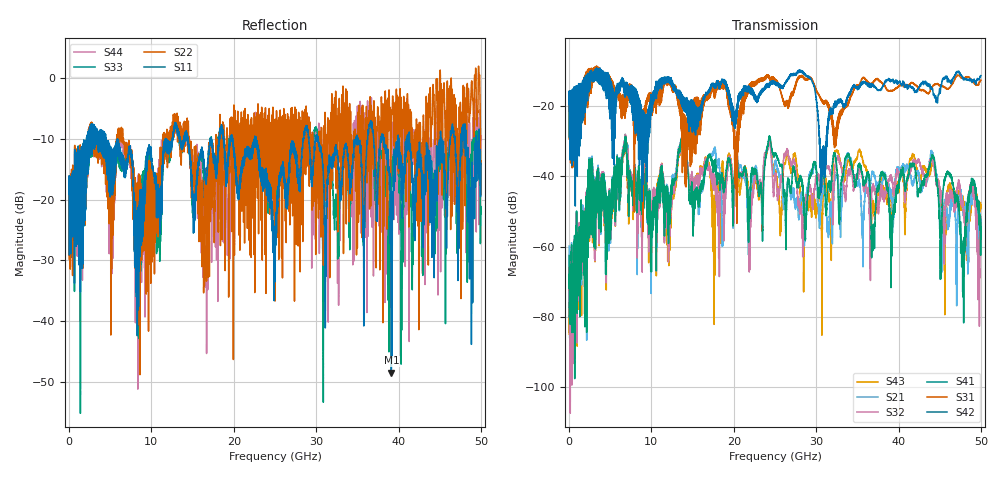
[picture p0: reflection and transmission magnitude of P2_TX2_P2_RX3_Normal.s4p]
!Keysight Technologies,N5225B,MY57041031,A.13.20.10
!Date: Friday, May 31, 2019 11:30:48
!Correction: S11(Full 4 Port(1,2,3,4))
!S12(Full 4 Port(1,2,3,4))
!S13(Full 4 Port(1,2,3,4))
!S14(Full 4 Port(1,2,3,4))
!S21(Full 4 Port(1,2,3,4))
!S22(Full 4 Port(1,2,3,4))
!S23(Full 4 Port(1,2,3,4))
!S24(Full 4 Port(1,2,3,4))
!S31(Full 4 Port(1,2,3,4))
!S32(Full 4 Port(1,2,3,4))
!S33(Full 4 Port(1,2,3,4))
!S34(Full 4 Port(1,2,3,4))
!S41(Full 4 Port(1,2,3,4))
!S42(Full 4 Port(1,2,3,4))
!S43(Full 4 Port(1,2,3,4))
!S44(Full 4 Port(1,2,3,4))
!S4P File: Measurements: <S11,S12,S13,S14>,
!<S21,S22,S23,S24>,
!<S31,S32,S33,S34>,
!<S41,S42,S43,S44>:
# Hz S  dB  R 50.0
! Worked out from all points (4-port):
!   5000 points, 10 MHz to 50 GHz, reference 50 ohm
!   strongest paths, dB at 10 MHz, 12.51 GHz, 25.01 GHz, 37.51 GHz, 50 GHz:
!     S42: -19.4, -14.3, -13.2, -15.4, -11.3
!     S31: -19.3, -14.9, -13.0, -12.4, -12.6
!     S41: -62.6, -42.6, -33.4, -42.7, -56.5
!     S32: -75.2, -44.8, -40.0, -49.1, -51.6
!     S21: -59.8, -42.2, -36.1, -42.0, -53.5
!     S43: -72.5, -45.7, -38.4, -44.4, -48.1
!   lowest |S11| = -48.4 dB at 39.13 GHz (marker M1), VSWR 1.01, Z = 49.9 + j0.354 ohm
!   |S11| at or under -10 dB: 4.481 GHz to 11.72 GHz (7.238 GHz wide, 89.4 % of centre); 22.72 GHz to 28.43 GHz (5.702 GHz wide, 22.3 % of centre); 30.26 GHz to 34.82 GHz (4.557 GHz wide, 14 % of centre)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
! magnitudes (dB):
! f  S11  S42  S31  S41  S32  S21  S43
! 10 MHz  -19.1  -19.4  -19.3  -62.6  -75.2  -59.8  -72.5
! 6.75 GHz  -16.0  -15.2  -22.3  -31.5  -30.5  -30.6  -31.5
! 10.06 GHz  -14.6  -19.8  -17.7  -57.5  -52.8  -54.8  -54.4
! 28.15 GHz  -15.5  -9.9  -11.4  -40.2  -48.4  -46.5  -47.3
! 30.79 GHz  -14.8  -32.0  -18.9  -37.8  -41.9  -44.7  -50.8
! 39.13 GHz  -48.4  -12.7  -15.6  -56.5  -40.6  -46.4  -48.1
! 50 GHz  -14.1  -11.3  -12.6  -56.5  -51.6  -53.5  -48.1
